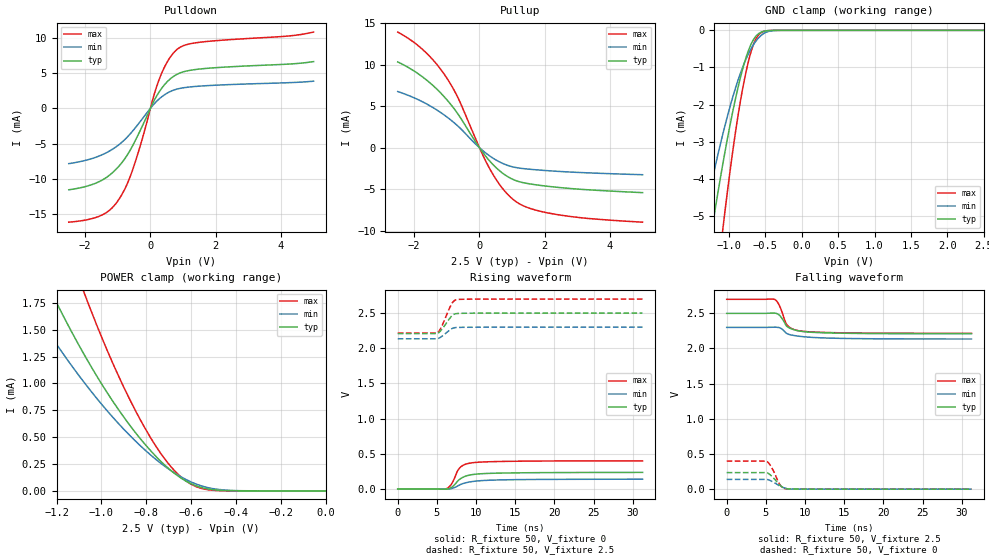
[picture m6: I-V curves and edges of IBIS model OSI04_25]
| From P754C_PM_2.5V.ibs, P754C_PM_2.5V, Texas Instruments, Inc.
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[Model]   OSI04_25
Model_type  3-state
Enable   Active-Low
Vref =   1.25
Rref =   50
Cref =   15p
Vmeas =   1.25
| variable   typ   min   max
C_comp   0.96pF   0.63pF   1.20pF
| C_pullup   1.20pF   0.63pF   1.60pF
| C_pulldown   1.13pF   0.75pF   1.42pF
| C_tri-state   0.96pF   0.63pF   1.20pF
[Temperature Range]   40   125   -40
| Ambient temperature   25   110   -40
[Voltage range]   2.5   2.3   2.7
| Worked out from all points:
|   slope of the pulldown table from 0 to 0.375 V, typ, clamps not added: 124 ohm
|   slope of the pullup table from 0 to 0.375 V, typ, clamps not added: 200 ohm
|   GND clamp passes 1 mA (typ) near -0.81 V on its own axis
|   POWER clamp passes 1 mA (typ) near -1.00 V on its own axis
|   rising waveform, R_fixture 50, V_fixture 0: 20-80 % time 1.69ns typ, 2.51ns min, 1.2ns max; typ from 0.001 V to 0.236 V
|   falling waveform, R_fixture 50, V_fixture 2.5: 20-80 % time 1.61ns typ, 2.58ns min, 1.13ns max; typ from 2.5 V to 2.21 V
|   rising waveform, R_fixture 50, V_fixture 2.5: 20-80 % time 1.14ns typ, 1.14ns min, 1.13ns max; typ from 2.21 V to 2.5 V
|   falling waveform, R_fixture 50, V_fixture 0: 20-80 % time 1.19ns typ, 1.33ns min, 1.03ns max; typ from 0.236 V to 0.001 V
[GND Clamp]
| OSI04_25
|   Voltage   I(typ)   I(min)   I(max)
-2.5V     -25.13mA   -18.8mA    -34.93mA
-1.375V   -7.204mA   -5.39mA    -10.6mA
-1.35V    -6.868mA   -5.146mA   -10.12mA
-1.22V    -5.193mA   -3.937mA   -7.7mA
-1.08V    -3.548mA   -2.76mA    -5.28mA
-920mV    -1.926mA   -1.614mA   -2.867mA
-790mV    -888.6uA   -885.3uA   -1.347mA
-725mV    -505.2uA   -602.1uA   -775.6uA
-675mV    -290.6uA   -423uA     -443uA
-565mV    -55.9uA    -148uA     -72.32uA
-345mV    -541.1nA   -2.823uA   -320.9nA
2.5V      136.8pA    30.93nA    99.28pA
[POWER Clamp]
| OSI04_25
|   Voltage   I(typ)   I(min)   I(max)
-2.5V     9.813mA    7.22mA     13.88mA
-1.345V   2.395mA    1.835mA    3.527mA
-1.21V    1.793mA    1.395mA    2.631mA
-1.08V    1.28mA     1.017mA    1.86mA
-1.05V    1.171mA    936.9uA    1.696mA
-945mV    821uA      675.4uA    1.167mA
-825mV    481.7uA    417.3uA    655.4uA
-735mV    274.5uA    256.5uA    347uA
-640mV    112.4uA    124.5uA    120uA
-575mV    45.32uA    61.76uA    37.21uA
-505mV    11.93uA    21.92uA    6.156uA
-31.11fV  136.8pA    628.5pA    110.9pA
[Pulldown]
| OSI04_25
|   Voltage   I(typ)   I(min)   I(max)
-2.5V     -11.57mA   -7.856mA   -16.16mA
-1.485V   -10.21mA   -6.607mA   -15.15mA
-1.19V    -9.255mA   -5.893mA   -14.21mA
-930mV    -8.036mA   -5.041mA   -12.68mA
-705mV    -6.615mA   -4.071mA   -10.68mA
-495mV    -4.875mA   -2.959mA   -8.057mA
110mV     1.045mA    594.5uA    1.862mA
290mV     2.466mA    1.409mA    4.341mA
555mV     3.947mA    2.252mA    6.873mA
840mV     4.877mA    2.754mA    8.438mA
1.515V    5.573mA    3.146mA    9.371mA
5V        6.623mA    3.846mA    10.81mA
[Pullup]
| OSI04_25
|   Voltage   I(typ)   I(min)   I(max)
-2.5V     10.32mA    6.756mA    13.91mA
-1.72V    8.457mA    5.479mA    11.75mA
-1.385V   7.353mA    4.739mA    10.41mA
-1.075V   6.12mA     3.927mA    8.838mA
-650mV    4.024mA    2.575mA    5.968mA
40mV      -208.3uA   -129.3uA   -323.1uA
330mV     -1.663mA   -1.033mA   -2.619mA
695mV     -3.023mA   -1.862mA   -4.83mA
1.07V     -3.891mA   -2.356mA   -6.343mA
1.53V     -4.351mA   -2.594mA   -7.28mA
2.31V     -4.743mA   -2.829mA   -8.009mA
5V        -5.415mA   -3.259mA   -8.973mA
[Ramp]
| OSI04_25
| variable   typ   min   max
dV/dt_r   0.14/1.75E-09   0.08/2.54E-09   0.24/1.20E-09
dV/dt_f   0.18/1.64E-09   0.10/2.58E-09   0.28/1.13E-09
R_load = 50
[Rising Waveform]
| OSI04_25
R_fixture =   50
C_fixture =   0
L_fixture =   0
V_fixture =   0
V_fixture_min = 0
V_fixture_max = 0
|   Time   V(typ)   V(min)   V(max)
0s        627uV      473.6uV    826.3uV
6.265ns   -877.4uV   -2.131mV   6.116mV
6.885ns   24.91mV    7.266mV    75.05mV
7.195ns   53.69mV    18.61mV    140.3mV
7.61ns    107.6mV    40.81mV    252mV
7.955ns   142.3mV    60.76mV    304.9mV
8.635ns   181.7mV    87.44mV    351.2mV
9.685ns   207.5mV    108.6mV    375mV
14.99ns   229.3mV    133mV      394.5mV
31.25ns   235.8mV    139.2mV    400mV
[Falling Waveform]
| OSI04_25
R_fixture =   50
C_fixture =   0
L_fixture =   0
V_fixture =   2.5
V_fixture_min = 2.3
V_fixture_max = 2.7
|   Time   V(typ)   V(min)   V(max)
0s        2.499V     2.3V       2.699V
6.13ns    2.502V     2.302V     2.698V
6.43ns    2.495V     2.301V     2.667V
6.74ns    2.472V     2.296V     2.607V
7.5ns     2.344V     2.229V     2.376V
7.715ns   2.312V     2.211V     2.334V
8.405ns   2.274V     2.189V     2.277V
9.475ns   2.245V     2.171V     2.248V
15.55ns   2.216V     2.142V     2.221V
31.25ns   2.209V     2.135V     2.217V
[Rising Waveform]
| OSI04_25
R_fixture =   50
C_fixture =   0
L_fixture =   0
V_fixture =   2.5
V_fixture_min = 2.3
V_fixture_max = 2.7
|   Time   V(typ)   V(min)   V(max)
0s        2.209V     2.135V     2.217V
5.075ns   2.21V      2.135V     2.22V
5.29ns    2.226V     2.145V     2.247V
5.64ns    2.27V      2.17V      2.318V
6.405ns   2.389V     2.238V     2.519V
6.885ns   2.46V      2.277V     2.633V
7.24ns    2.486V     2.291V     2.677V
7.62ns    2.494V     2.296V     2.692V
10.98ns   2.499V     2.299V     2.698V
31.25ns   2.499V     2.3V       2.699V
[Falling Waveform]
| OSI04_25
R_fixture =   50
C_fixture =   0
L_fixture =   0
V_fixture =   0
V_fixture_min = 0
V_fixture_max = 0
|   Time   V(typ)   V(min)   V(max)
0s        236.2mV    139.5mV    400.1mV
5.1ns     235.3mV    139.4mV    397.8mV
5.385ns   219.3mV    131.4mV    367.7mV
5.735ns   186.2mV    113.9mV    307.9mV
6.13ns    140.8mV    89.38mV    223.1mV
6.585ns   82.16mV    58.58mV    104.1mV
6.815ns   55.51mV    43.52mV    61.15mV
7.18ns    25.18mV    24.88mV    19.87mV
7.61ns    6.689mV    11.04mV    5.68mV
31.25ns   642.8uV    483.1uV    833.5uV
